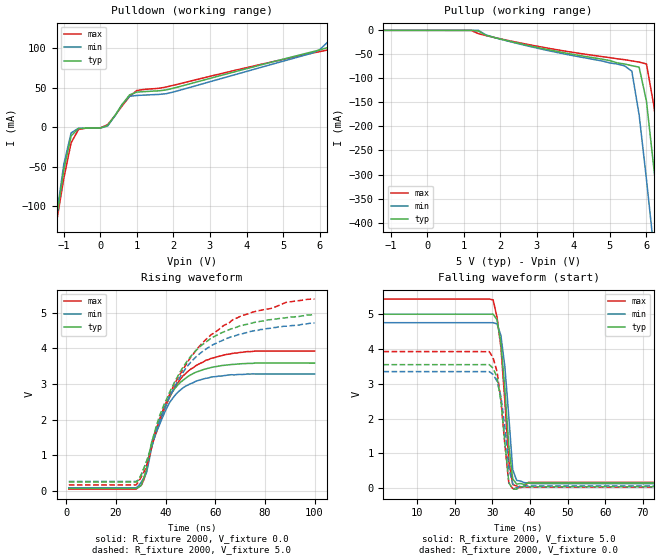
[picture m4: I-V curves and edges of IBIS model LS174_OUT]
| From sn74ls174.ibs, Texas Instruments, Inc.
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|   Model LS174_OUT
[Model]   LS174_OUT
Model_type  Output
Polarity   Inverting
Vmeas = 1.3v
Cref = 15pf
Rref = 2000
| variable   typ   min   max
C_comp   5.60pf   4.20pf   7.00pf
[Temperature Range]   25   0   70
[Voltage Range]   5.00   4.75   5.25
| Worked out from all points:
|   slope of the pulldown table from 0 to 0.75 V, typ, clamps not added: 19.2 ohm
|   rising waveform, R_fixture 2000, V_fixture 0.0: 20-80 % time 11.1ns typ, 10.4ns min, 13ns max; typ from 0.072 V to 3.59 V
|   falling waveform, R_fixture 2000, V_fixture 5.0: 20-80 % time 2.09ns typ, 2.13ns min, 2.23ns max; typ from 4.99 V to 0.159 V
|   rising waveform, R_fixture 2000, V_fixture 5.0: 20-80 % time 19.5ns typ, 19.3ns min, 23.3ns max; typ from 0.251 V to 4.96 V
|   falling waveform, R_fixture 2000, V_fixture 0.0: 20-80 % time 2.1ns typ, 2.08ns min, 2.25ns max; typ from 3.54 V to 0.047 V
[Pulldown]
|   Voltage   I(typ)   I(min)   I(max)
-5V       -1.589A    -1.709A    -1.414A
-1.4V     -192.1mA   -193.6mA   -188.6mA
-1.2V     -115.5mA   -112.3mA   -120.6mA
-1V       -53.99mA   -46.9mA    -64.64mA
-800mV    -11.05mA   -7.318mA   -19.73mA
-600mV    -1.763mA   -1.485mA   -3.076mA
200mV     2.253mA    1.434mA    3.279mA
1V        44.4mA     40.14mA    46.45mA
5.8V      95.44mA    93.83mA    93.73mA
6.8V      122.3mA    129.1mA    111.2mA
7.4V      141.4mA    147.8mA    130.7mA
10V       223.6mA    227.9mA    214.4mA
[Pullup]
|   Voltage   I(typ)   I(min)   I(max)
-5V       2.751uA    649.5nA    18.57uA
1.4V      -1.523mA   -61.48uA   -6.907mA
2.6V      -28.75mA   -29.78mA   -27.07mA
5.4V      -70.02mA   -73.84mA   -61.06mA
5.6V      -73.5mA    -85mA      -63.58mA
5.8V      -76.68mA   -175.9mA   -66.03mA
6V        -147.2mA   -309.9mA   -69.96mA
6.2V      -285.1mA   -453mA     -155.4mA
6.4V      -418.1mA   -591.7mA   -267.9mA
6.6V      -548.4mA   -727.9mA   -387.4mA
6.8V      -675.6mA   -862.2mA   -504.6mA
10V       -2.654A    -3.011A    -2.322A
[Ramp]
| variable   typ   min   max
dV/dt_r   2.034E+00/1.080E-08   1.836E+00/1.002E-08   2.280E+00/1.283E-08
dV/dt_f   2.934E+00/1.914E-09   2.772E+00/1.928E-09   3.096E+00/1.913E-09
R_load = 2000
[Rising Waveform]
R_fixture = 2000
V_fixture = 0.0
V_fixture_min = 0.0
V_fixture_max = 0.0
C_fixture = 0pf
L_fixture = 0nH
|   Time   V(typ)   V(min)   V(max)
1.042ns   72.27mV    90.3mV     51.69mV
28.13ns   72.27mV    90.3mV     51.69mV
30.21ns   164.2mV    250.9mV    156.7mV
32.29ns   611.8mV    509.9mV    537.2mV
34.38ns   1.366V     1.222V     1.238V
40.63ns   2.517V     2.35V      2.475V
45.83ns   3.041V     2.825V     3.127V
52.08ns   3.329V     3.076V     3.512V
72.92ns   3.579V     3.283V     3.913V
100ns     3.588V     3.283V     3.925V
[Falling Waveform]
R_fixture = 2000
V_fixture = 5.0
V_fixture_min = 4.75
V_fixture_max = 5.25
C_fixture = 0pf
L_fixture = 0nH
|   Time   V(typ)   V(min)   V(max)
1.042ns   4.99V      4.746V     5.423V
30.21ns   4.99V      4.746V     5.4V
31.25ns   4.829V     4.713V     4.901V
32.29ns   4.157V     4.376V     4.03V
33.33ns   2.854V     3.489V     2.508V
34.38ns   1.221V     2.069V     784.3mV
35.42ns   274.2mV    538.2mV    109.7mV
36.46ns   122.2mV    229.3mV    69.28mV
40.63ns   158.8mV    132.9mV    171.3mV
100ns     158.8mV    132.9mV    171.3mV
[Rising Waveform]
R_fixture = 2000
V_fixture = 5.0
V_fixture_min = 4.75
V_fixture_max = 5.25
C_fixture = 0pf
L_fixture = 0nH
|   Time   V(typ)   V(min)   V(max)
1.042ns   250.6mV    268.6mV    170mV
28.13ns   250.6mV    268.6mV    169.8mV
29.17ns   315.7mV    309mV      267.5mV
32.29ns   825.2mV    811.6mV    698.7mV
37.5ns    2.09V      1.956V     1.987V
41.67ns   2.776V     2.651V     2.72V
47.92ns   3.564V     3.416V     3.509V
54.17ns   4.07V      3.878V     4.102V
70.83ns   4.642V     4.408V     4.928V
100ns     4.955V     4.713V     5.385V
[Falling Waveform]
R_fixture = 2000
V_fixture = 0.0
V_fixture_min = 0.0
V_fixture_max = 0.0
C_fixture = 0pf
L_fixture = 0nH
|   Time   V(typ)   V(min)   V(max)
1.042ns   3.544V     3.345V     3.918V
29.17ns   3.546V     3.345V     3.92V
30.21ns   3.443V     3.264V     3.738V
31.25ns   3.179V     3.072V     3.348V
32.29ns   2.492V     2.638V     2.526V
33.33ns   1.321V     1.76V      1.263V
34.38ns   167.8mV    578.5mV    157mV
35.42ns   -21.27mV   131mV      -5.087mV
36.46ns   -22.49mV   13.17mV    -5.918mV
100ns     47.38mV    69.06mV    35.94mV
